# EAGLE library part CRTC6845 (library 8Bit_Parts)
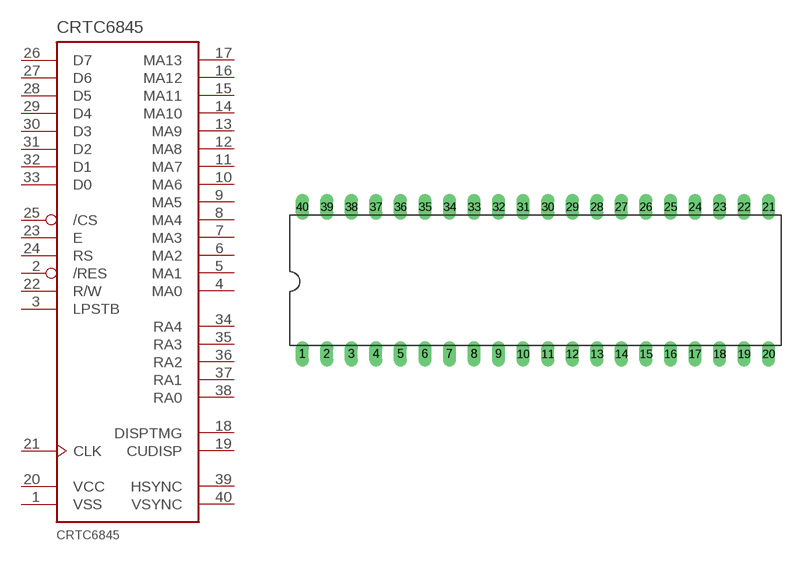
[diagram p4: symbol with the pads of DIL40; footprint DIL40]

Designator prefix IC

## CRTC6845  [DIL40]
1  VSS  pwr
2  /RES  in
3  LPSTB  in
4  MA0  out
5  MA1  out
6  MA2  out
7  MA3  out
8  MA4  out
9  MA5  out
10  MA6  out
11  MA7  out
12  MA8  out
13  MA9  out
14  MA10  out
15  MA11  out
16  MA12  out
17  MA13  out
18  DISPTMG  out
19  CUDISP  out
20  VCC  pwr
21  CLK  in
22  R/W  in
23  E  in
24  RS  in
25  /CS  in
26  D7
27  D6
28  D5
29  D4
30  D3
31  D2
32  D1
33  D0
34  RA4  out
35  RA3  out
36  RA2  out
37  RA1  out
38  RA0  out
39  HSYNC  out
40  VSYNC  out

## Footprint DIL40 (pad centres in mm)
Dual In Line Package
drill 0.813 long: 1 -24.13,-7.62; 2 -21.59,-7.62; 3 -19.05,-7.62; 4 -16.51,-7.62; 5 -13.97,-7.62; 6 -11.43,-7.62; 7 -8.89,-7.62; 8 -6.35,-7.62; 9 -3.81,-7.62; 10 -1.27,-7.62; 11 1.27,-7.62; 12 3.81,-7.62; 13 6.35,-7.62; 14 8.89,-7.62; 15 11.43,-7.62; 16 13.97,-7.62; 17 16.51,-7.62; 18 19.05,-7.62; 19 21.59,-7.62; 20 24.13,-7.62; 21 24.13,7.62; 22 21.59,7.62; 23 19.05,7.62; 24 16.51,7.62; 25 13.97,7.62; 26 11.43,7.62; 27 8.89,7.62; 28 6.35,7.62; 29 3.81,7.62; 30 1.27,7.62; 31 -1.27,7.62; 32 -3.81,7.62; 33 -6.35,7.62; 34 -8.89,7.62; 35 -11.43,7.62; 36 -13.97,7.62; 37 -16.51,7.62; 38 -19.05,7.62; 39 -21.59,7.62; 40 -24.13,7.62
